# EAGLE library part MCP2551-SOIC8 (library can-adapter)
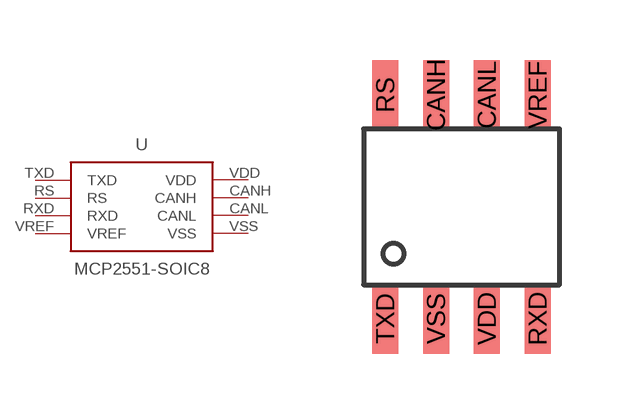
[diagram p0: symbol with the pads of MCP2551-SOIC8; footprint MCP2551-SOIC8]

Designator prefix -

## MCP2551-SOIC8  [MCP2551-SOIC8]
CANH  CANH
CANL  CANL
RS  RS  in
RXD  RXD  out
TXD  TXD  in
VDD  VDD  pwr
VREF  VREF  out
VSS  VSS  pwr

## Footprint MCP2551-SOIC8 (pad centres in mm)
smd 0.65 x 1.75: CANH -0.635,2.8; CANL 0.635,2.8; RS -1.905,2.8; RXD 1.905,-2.8; TXD -1.905,-2.8; VDD 0.635,-2.8; VREF 1.905,2.8; VSS -0.635,-2.8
